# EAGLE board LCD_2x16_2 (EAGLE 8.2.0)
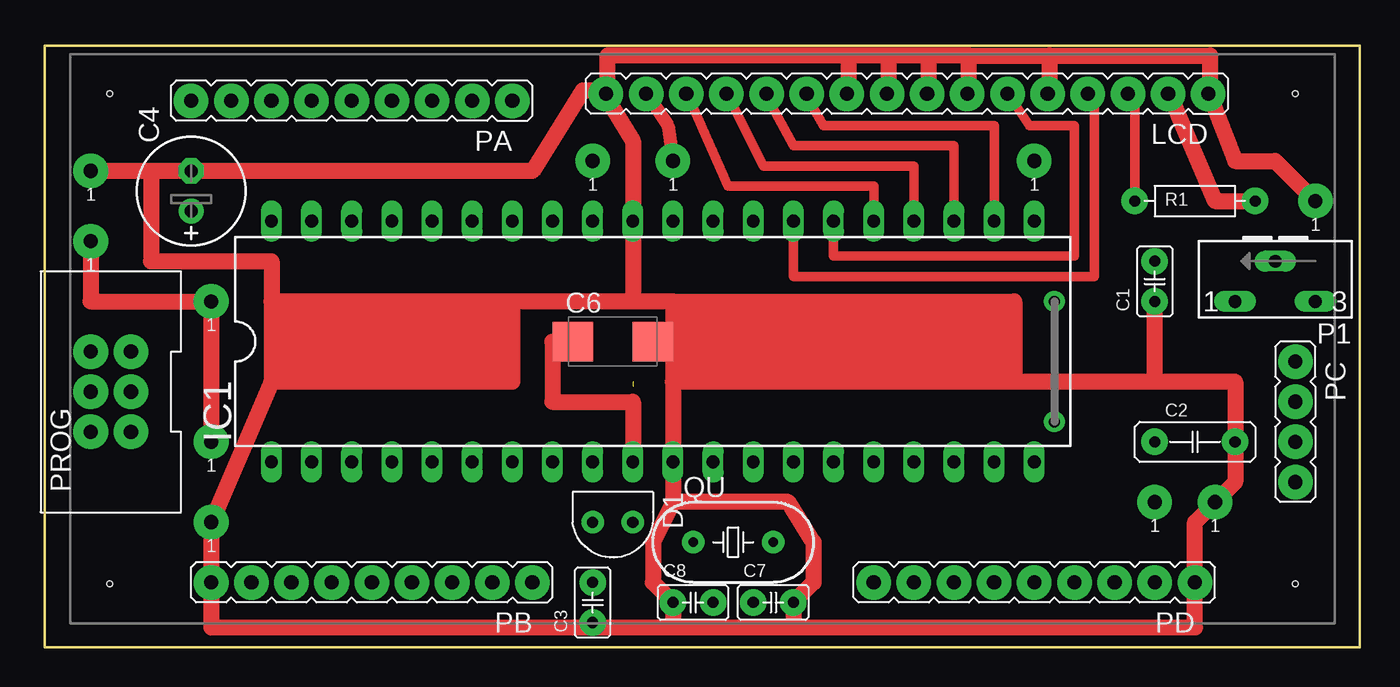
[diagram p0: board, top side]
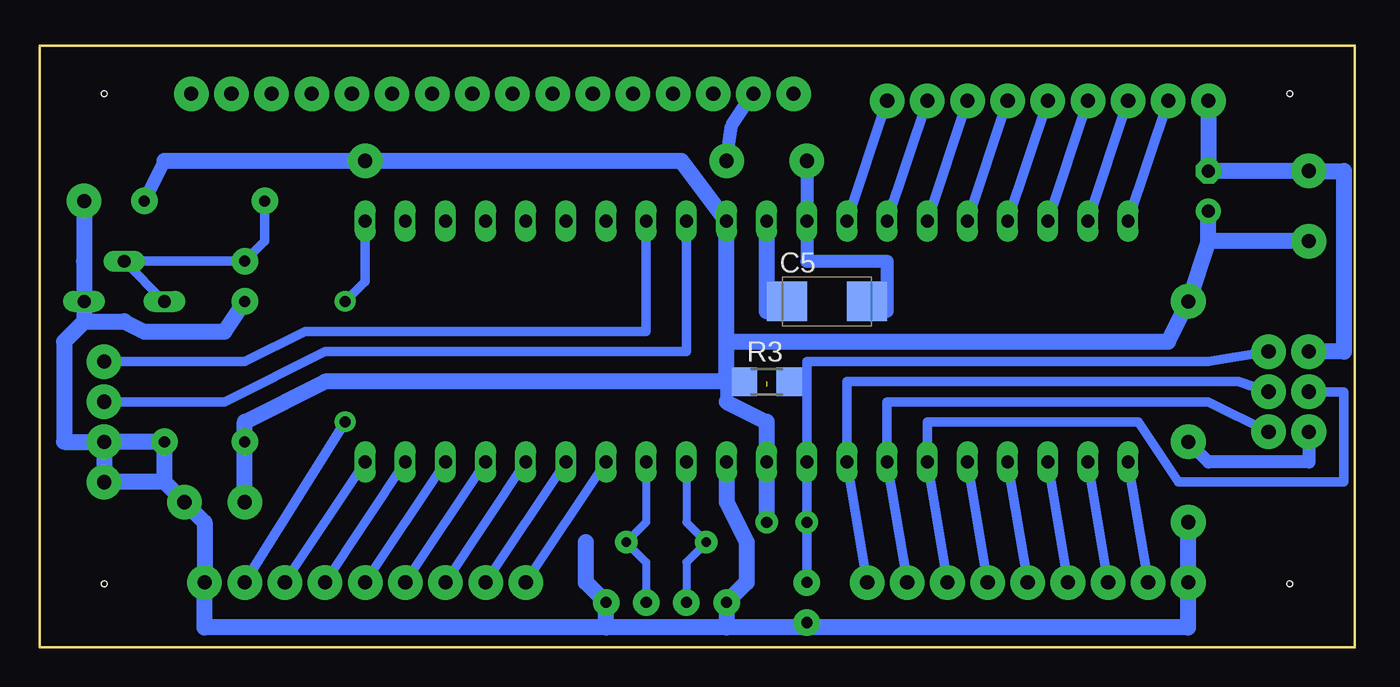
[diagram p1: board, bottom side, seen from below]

Size 83.2 x 38.06 mm. Coordinates in mm from the lower left corner, seen from the top.
Outline: 0,0 83.2,0 83.2,38.06 0,38.06 0,0
Copper layers (1*16): Top 0.035mm / dielectric 1.5mm / Bottom 0.035mm
Design rules "default": minimum track width 10mil, minimum drill 24mil, track to track 8mil, track to pad 8mil, pad to pad 8mil, via to via 8mil, smd to smd 8mil, copper to edge 40mil, drill to drill 8mil, minimum pad ring 10mil, minimum via ring 8mil, stop-mask expansion 4mil, vias tented up to drill 0mil, thermal gap 10mil
Holes 0.35 mm at 4.1,4.03 79.1,4.03 4.1,35.03 79.1,35.03

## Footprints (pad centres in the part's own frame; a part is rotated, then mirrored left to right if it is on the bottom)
C-2.5 = drill 0.7 pad 1.676: 1 -1.27,0; 2 1.27,0
C-5 = drill 0.7 pad 1.676: 1 -2.54,0; 2 2.54,0
E2,5-7 = drill 0.813 pad 1.6: + -1.27,0 | drill 0.813 pad 1.6 octagon: - 1.27,0
C/6032-28R = smd 2.55 x 2.5: + 2.525,0; - -2.525,0
TO92-D = drill 0.7 pad 1.422: A 1.27,-1.27; K 1.27,1.27
1-POL. = drill 0.9 pad 2.184: 1 0,0
DIL40 = drill 0.813 long: 1 -24.13,-7.62; 2 -21.59,-7.62; 3 -19.05,-7.62; 4 -16.51,-7.62; 5 -13.97,-7.62; 6 -11.43,-7.62; 7 -8.89,-7.62; 8 -6.35,-7.62; 9 -3.81,-7.62; 10 -1.27,-7.62; 11 1.27,-7.62; 12 3.81,-7.62; 13 6.35,-7.62; 14 8.89,-7.62; 15 11.43,-7.62; 16 13.97,-7.62; 17 16.51,-7.62; 18 19.05,-7.62; 19 21.59,-7.62; 20 24.13,-7.62; 21 24.13,7.62; 22 21.59,7.62; 23 19.05,7.62; 24 16.51,7.62; 25 13.97,7.62; 26 11.43,7.62; 27 8.89,7.62; 28 6.35,7.62; 29 3.81,7.62; 30 1.27,7.62; 31 -1.27,7.62; 32 -3.81,7.62; 33 -6.35,7.62; 34 -8.89,7.62; 35 -11.43,7.62; 36 -13.97,7.62; 37 -16.51,7.62; 38 -19.05,7.62; 39 -21.59,7.62; 40 -24.13,7.62
16-POL. = drill 0.9 pad 2.184: 1 0,0; 2 2.54,0; 3 5.08,0; 4 7.62,0; 5 10.16,0; 6 12.7,0; 7 15.24,0; 8 17.78,0; 9 20.32,0; 10 22.86,0; 11 25.4,0; 12 27.94,0; 13 30.48,0; 14 33.02,0; 15 35.56,0; 16 38.1,0
S63X = drill 0.813 long: A 2.54,0; E -2.54,0; S 0,-2.54
9-POL. = drill 0.9 pad 2.184: 1 0,0; 2 2.54,0; 3 5.08,0; 4 7.62,0; 5 10.16,0; 6 12.7,0; 7 15.24,0; 8 17.78,0; 9 20.32,0
4-POL. = drill 0.9 pad 2.184: 1 0,0; 2 2.54,0; 3 5.08,0; 4 7.62,0
2X3-POL. = drill 0.9 pad 2.184: 1 0,0; 2 0,2.54; 3 2.54,0; 4 2.54,2.54; 5 5.08,0; 6 5.08,2.54
QUARZ_49V = drill 0.6 pad 1.422: P1 -2.54,0; P2 2.54,0
R-7.5 = drill 0.7 pad 1.676: 1 -2.54,0; 2 5.08,0
R1206 = smd 1.6 x 1.803: 1 -1.422,0; 2 1.422,0

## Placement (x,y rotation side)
C1  [C-2.5]  70.22,23.16 90 top
C2  [C-5]  72.76,13 0 top
C3  [C-2.5]  34.66,2.84 90 top
C4  [E2,5-7]  9.26,28.88 90 top
C5  [C/6032-28R]  33.39,21.89 0 bottom
C6  [C/6032-28R]  35.93,19.35 0 top
C7  [C-2.5]  46.09,2.84 0 top
C8  [C-2.5]  41.01,2.84 0 top
D1  [TO92-D]  35.93,9.19 270 top
E$1  [1-POL.]  80.38,28.24 0 top
E$2  [1-POL.]  34.66,30.78 0 top
E$5  [1-POL.]  70.22,9.19 0 top
E$6  [1-POL.]  10.53,13 0 top
E$7  [1-POL.]  10.53,21.89 0 top
E$8  [1-POL.]  74.03,9.19 0 top
E$9  [1-POL.]  10.53,7.92 0 top
E$10  [1-POL.]  39.74,30.78 0 top
E$11  [1-POL.]  62.6,30.78 0 top
E$12  [1-POL.]  2.91,30.14 0 top
E$13  [1-POL.]  2.91,25.7 0 top
IC1  [DIL40]  38.47,19.35 0 top
LCD  [16-POL.]  73.6,35.03 180 top
P1  [S63X]  77.84,21.89 180 top
PA  [9-POL.]  29.58,34.59 180 top
PB  [9-POL.]  30.85,4.11 180 top
PC  [4-POL.]  79.11,18.08 270 top
PD  [9-POL.]  72.76,4.11 180 top
PROG  [2X3-POL.]  5.45,13.63 90 top
QU  [QUARZ_49V]  43.55,6.65 0 top
R1  [R-7.5]  71.49,28.24 0 top
R3  [R1206]  37.2,16.81 0 bottom

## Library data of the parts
C1-C3 C7 C8 R1 = 1_Passive
C4-C6 R3 = rcl
D1 = 1_Aktive
E$1 E$2 E$5-E$13 LCD PA PB PC PD PROG = 1_Stiftleiste
IC1 = atmel
P1 = pot
QU = 1_Quarz

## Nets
GND: C1.1 C2.2 C3.1 C4.- C7.2 C8.1 E$1.1 E$8.1 E$9.1 E$12.1 IC1.11 IC1.31 PB.9 PC.3 PC.4 PD.1 PROG.6
KONTR: C1.2 P1.A P1.S R1.1
MISO: IC1.7 PB.2 PROG.1
MOSI: IC1.6 PB.3 PROG.4
REF: E$2.1 IC1.32
RESET: C3.2 D1.A IC1.9 PROG.5
S$1: IC1.28 PC.1
S$2: C8.2 IC1.12 QU.P1
S$4: IC1.27
S$5: IC1.22
S$6: IC1.23
S$7: IC1.24
S$8: IC1.25
S$9: IC1.29 PC.2
S$10: IC1.40
S$11: IC1.39
S$12: IC1.38
S$13: IC1.37
S$14: IC1.36
S$15: IC1.35
S$16: IC1.34
S$17: IC1.33
S$18: C7.1 IC1.13 QU.P2
S$19: E$10.1
S$20: IC1.26
S$23: IC1.14 PD.9
S$24: IC1.15 PD.8
S$25: IC1.16 PD.7
S$26: IC1.17 PD.6
S$27: IC1.18 PD.5
S$28: IC1.19 PD.4
S$29: IC1.20 PD.3
S$30: IC1.21 PD.2
S$31: IC1.5 PB.4
S$32: IC1.4 PB.5
S$33: IC1.3 PB.6
S$34: IC1.2 PB.7
S$35: IC1.1 PB.8
SCK: IC1.8 PB.1 PROG.3
VCC: C4.+ D1.K E$5.1 E$6.1 E$7.1 E$13.1 IC1.10 IC1.30 PROG.2 R1.2

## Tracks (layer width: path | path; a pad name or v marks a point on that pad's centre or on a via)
GND
  Top 0.813: 35.3,35.23 35.61,34.91
  Top 1.016: 58.47,35.23 58.47,37.45 | 58.47,37.45 63.55,37.45 | 63.55,37.45 73.71,37.45 73.71,34.91 75.3,30.78 77.84,30.78 E$1.1 | 58.47,37.45 55.93,37.45 | 55.93,37.45 53.39,37.45 | 53.39,37.45 50.85,37.45 | 50.85,37.45 50.85,35.23 | 53.39,35.23 53.39,37.45 | 55.93,35.23 55.93,37.45 | 63.55,37.45 63.55,35.23 | 39.74,21.89 39.74,16.81 | 39.74,16.81 IC1.11 39.74,9.19 | 50.85,37.45 35.61,37.45 35.61,34.91 | 39.74,16.81 61.33,16.81 | 61.33,16.81 70.22,16.81 | 70.22,16.81 75.3,16.81 C2.2 75.3,10.46 E$8.1 72.76,7.92 72.76,1.25 47.36,1.25 | 6.72,30.14 30.85,30.14 34.02,35.23 35.3,35.23 37.2,32.05 IC1.31 37.2,21.89 | 39.74,21.89 37.2,21.89 | 37.2,21.89 29.58,21.89 | 29.58,21.89 14.34,21.89 | 6.72,30.14 E$12.1 | 6.72,30.14 6.72,24.43 14.34,24.43 14.34,21.89 | 14.34,21.89 14.34,16.81 | 14.34,16.81 E$9.1 PB.9 10.53,1.25 39.74,1.25 | 70.22,16.81 C1.1 | 39.74,1.25 47.36,1.25 | 39.74,9.19 38.47,6.65 38.47,4.11 C8.1 39.74,1.25 | 47.36,1.25 C7.2 48.63,4.11 48.63,6.65 47.04,9.19 39.74,9.19 | 39.74,21.89 61.33,21.89 61.33,16.81 | 14.34,16.81 29.58,16.81 29.58,21.89
  Bottom 0.508: 80.38,21.89 80.38,24.43 | C3.1 34.66,1.25
  Bottom 1.016: E$1.1 80.38,24.43 80.38,20.62 | IC1.11 39.74,9.19 38.47,6.65 38.47,4.11 C8.1 39.74,1.25 | 39.74,1.25 47.36,1.25 | 47.36,1.25 C7.2 48.63,4.11 48.63,6.65 | 47.36,1.25 72.76,1.25 PD.1 72.76,7.92 E$8.1 75.3,10.46 | 80.38,20.62 81.65,19.35 81.65,13 PC.3 | PC.3 PC.4 75.3,10.46 | 75.3,10.46 C2.2 PC.3 | 39.74,1.25 34.66,1.25 10.53,1.25 PB.9 E$9.1 | 9.26,34.59 C4.- E$12.1 0.69,30.14 0.69,18.71 PROG.6 | IC1.31 37.2,21.26 | 80.38,20.62 77.84,20.62 76.57,19.98 71.49,19.98 C1.1
KONTR
  Top 0.61: R1.1 68.95,34.59 68.63,34.91
  Bottom 0.61: R1.1 68.95,25.7 C1.2 P1.S P1.A
MISO
  Bottom 0.61: PROG.1 9.26,15.54 29.58,15.54 IC1.7 PB.2
MOSI
  Bottom 0.61: PROG.4 0.69,16.18 0.69,10.46 11.16,10.46 13.71,14.27 27.04,14.27 IC1.6 PB.3
REF
  Bottom 0.813: E$2.1 IC1.32 34.66,24.43 29.58,24.43 29.58,21.26
RESET
  Bottom 0.61: PROG.5 9.26,18.08 34.66,18.08 IC1.9 D1.A C3.2
S$1
  Bottom 0.61: IC1.28 44.82,19.98 66.41,19.98 70.22,18.08 PC.1
S$2
  Bottom 0.508: IC1.12 42.28,7.92 QU.P1 42.28,5.38 C8.2
S$4
  Top 0.61: 66.09,34.91 66.41,34.59 66.41,23.48 47.36,23.48 IC1.27
S$5
  Top 0.61: 48,35.23 49.27,33 60.06,33 IC1.22
S$6
  Top 0.61: 45.45,35.23 47.36,31.73 57.52,31.73 IC1.23
S$7
  Top 0.61: 43.23,34.91 45.45,30.46 54.98,30.46 IC1.24
S$8
  Top 0.61: 40.69,34.91 43.23,29.19 52.44,29.19 IC1.25
S$9
  Bottom 0.61: IC1.29 42.28,18.71 65.14,18.71 71.49,15.54 PC.2
S$10
  Bottom 0.61: 11.8,34.59 IC1.40
S$11
  Bottom 0.61: 14.34,34.59 IC1.39
S$12
  Bottom 0.61: 16.88,34.59 IC1.38
S$13
  Bottom 0.61: 19.42,34.59 IC1.37
S$14
  Bottom 0.61: 21.96,34.59 IC1.36
S$15
  Bottom 0.61: 24.5,34.59 IC1.35
S$16
  Bottom 0.61: 27.04,34.59 IC1.34
S$17
  Bottom 0.61: 29.58,34.59 IC1.33
S$18
  Bottom 0.508: IC1.13 44.82,7.92 QU.P2 44.82,5.38 C7.1
S$19
  Top 0.813: 38.15,34.91 39.42,33 E$10.1
  Bottom 0.813: E$10.1 39.42,33 38.15,34.91
S$20
  Top 0.61: 61.01,34.91 62.28,33 65.14,33 65.14,24.75 49.9,24.75 IC1.26
S$21
  Top 2.54: 41.01,18.08 60.06,18.08 60.06,20.62 41.01,20.62 41.01,18.08
S$22
  Top 2.54: 15.61,20.62 28.31,20.62 28.31,18.08 15.61,18.08 15.61,20.62
S$23
  Bottom 0.61: IC1.14 PD.9
S$24
  Bottom 0.61: IC1.15 PD.8
S$25
  Bottom 0.61: IC1.16 PD.7
S$26
  Bottom 0.61: IC1.17 PD.6
S$27
  Bottom 0.61: IC1.18 PD.5
S$28
  Bottom 0.61: IC1.19 PD.4
S$29
  Bottom 0.61: IC1.20 PD.3
S$30  (via drill 0.7 pad 1.3)
  Bottom 0.61: v63.87,14.27 PD.2 | IC1.21 62.6,23.16 v63.87,21.89
S$31
  Bottom 0.61: IC1.5 PB.4
S$32
  Bottom 0.61: IC1.4 PB.5
S$33
  Bottom 0.61: IC1.3 PB.6
S$34
  Bottom 0.61: IC1.2 PB.7
S$35
  Bottom 0.61: IC1.1 PB.8
S$39  (1 unrouted)
SCK
  Bottom 0.61: PB.1 IC1.8 32.12,16.81 7.36,16.81 PROG.3
VCC
  Top 1.016: E$6.1 E$7.1 2.91,21.89 E$13.1 | 32.12,19.35 32.12,15.54 37.2,15.54 IC1.10 | 71.17,34.91 74.03,28.24 R1.2
  Bottom 0.813: 75.3,30.78 R1.2 | PROG.2 2.91,11.73 9.26,11.73 E$6.1 | 39.74,16.81 39.74,15.54
  Bottom 1.016: 75.3,30.78 42.6,30.78 IC1.30 39.74,19.35 | 39.74,19.35 39.74,16.81 65.14,16.81 70.22,14.27 E$5.1 | 39.74,19.35 11.8,19.35 E$7.1 9.26,25.7 | E$13.1 9.26,25.7 | 9.26,25.7 C4.+ | 39.74,15.54 37.2,14.27 IC1.10 D1.K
